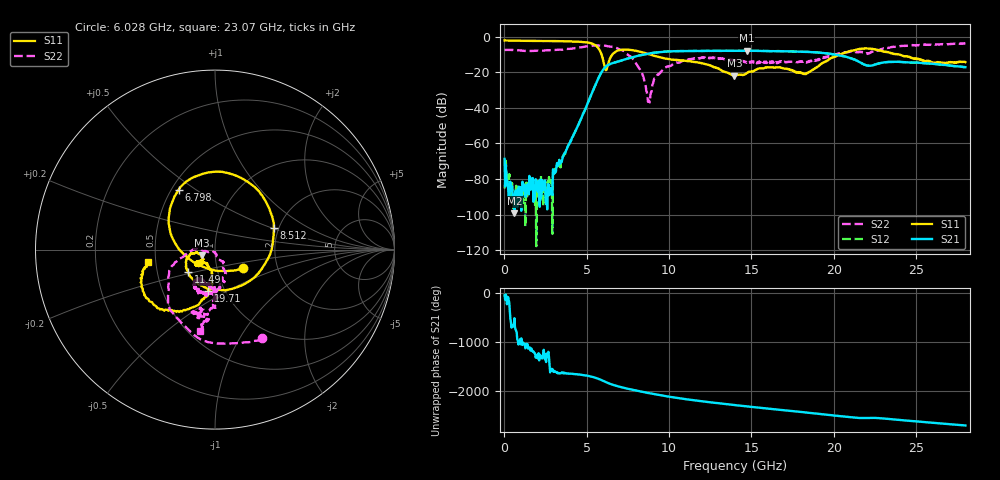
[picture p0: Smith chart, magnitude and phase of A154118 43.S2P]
!  2-Port S-parameters saved by WinCal
! VAR MeasName=S-Parameters (CALIBRATED_DATA) read from VNA (N5230A)
! VAR MeasDate=2015-9-10 14:37:47
! VAR NAME=A154118 43
! VAR FILENAME=A154118 43.S2P
! VAR DATE=2015-9-10 14:37:47
! VAR PHYS_PORTS=1,2
# Hz S DB R 50
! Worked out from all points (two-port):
!   801 points, 10 MHz to 28 GHz, reference 50 ohm
!   highest |S21| = -7.91 dB at 14.7 GHz (marker M1); lowest = -99.3 dB at 604.8 MHz (marker M2)
!   |S21| within 3 dB of the highest: 8.048 GHz to 20.57 GHz (12.52 GHz wide, 87.5 % of centre)
!   lowest |S11| = -21.9 dB at 13.97 GHz (marker M3), VSWR 1.18, Z = 43 - j2.66 ohm
!   |S11| at or under -10 dB: 5.896 GHz to 6.565 GHz (668.3 MHz wide, 10.7 % of centre); 8.822 GHz to 20.37 GHz (11.55 GHz wide, 79.1 % of centre); 23.95 GHz to end of sweep
!   |S22| runs from -37.0 to -3.7 dB; largest |S21 - S12| = 0.0075
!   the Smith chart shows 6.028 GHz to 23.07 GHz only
!   S11 on the Smith chart (normalised r, x): 6.028 GHz: 1.34, -0.29; 6.798 GHz: 0.54, +0.43; 8.512 GHz: 1.89, +0.52; 11.49 GHz: 0.72, -0.18; 19.71 GHz: 0.84, -0.40; 23.07 GHz: 0.45, -0.07
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1e7  -2.15 179.7  -68.68 -54.4  -85.28 -39.9  -7.49 179.8
2.549125e8  -2.18 176.2  -90.07 -145.1  -82.10 -151.6  -7.44 172.1
6.047875e8  -2.26 171.5  -99.26 -159.7  -96.26 124.9  -7.53 161.5
2.774012e9  -2.49 142.1  -85.06 177.0  -80.26 -81.8  -7.66 97.4
4.698325e9  -3.00 98.2  -45.10 125.6  -45.06 125.5  -5.95 13.0
5.608e9  -5.45 42.2  -25.37 57.4  -25.33 57.3  -4.93 -36.1
6.02785e9  -14.46 -33.1  -18.19 -1.5  -18.19 -1.6  -5.05 -62.0
6.797575e9  -8.17 121.3  -14.24 -98.7  -14.24 -98.7  -6.30 -105.3
7.812212e9  -7.64 60.1  -11.51 179.1  -11.53 179.0  -12.57 -162.2
8.511962e9  -9.12 20.1  -9.94 130.8  -9.92 130.9  -25.41 -174.6
8.791862e9  -9.95 2.3  -9.46 112.2  -9.41 112.0  -36.00 -90.9
9.351662e9  -11.36 -33.6  -8.81 77.7  -8.76 77.5  -21.41 -57.9
1.14859e10  -14.21 -140.6  -8.05 -31.1  -8.05 -31.7  -12.39 -91.1
1.397001e10  -21.86 -157.6  -7.95 -129.6  -7.95 -129.8  -13.29 -122.0
1.4005e10  -21.78 -157.3  -7.98 -130.8  -7.96 -131.2  -13.31 -122.7
1.470475e10  -20.59 -142.7  -7.91 -156.4  -7.88 -156.8  -14.69 -119.5
1.70839e10  -17.96 -146.5  -8.21 121.5  -8.21 121.2  -14.32 -111.8
1.869332e10  -18.73 -101.9  -8.71 65.5  -8.73 65.1  -13.15 -94.0
1.970796e10  -12.73 -99.3  -9.57 28.6  -9.52 28.2  -10.89 -90.5
2.306676e10  -8.42 -169.9  -14.44 -45.0  -14.53 -45.4  -6.69 -100.6
2.334666e10  -8.93 -171.5  -14.19 -53.3  -14.23 -54.3  -6.28 -103.9
2.8e10  -14.34 -154.5  -17.14 174.7  -17.19 174.7  -3.68 -138.4
